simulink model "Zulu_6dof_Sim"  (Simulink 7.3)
settings: Solver=ode45  StartTime=0.0  StopTime=315  RelTol=1e-4
InitFcn:
  | init
StopFcn:
  | pl
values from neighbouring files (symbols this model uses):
  accel = [-225, 0, 0]    [init.m]
  ch = 7.761    [init.m]
  d2r = pi/180    (= 0.0174532925199)    [init.m]    (also in pl.m; run.m; LQR_Des.m)
  Euler_0 = [0, 49.766, 0]*d2r    [init.m]
  h0 = 43031    [init.m]
  Ixxpr = ee*Zulu_Mass(:,2)    [init.m]
  Ixypr = ee*Zulu_Mass(:,5)    [init.m]
  Ixzpr = ee*Zulu_Mass(:,6)    [init.m]
  Iyypr = ee*Zulu_Mass(:,3)    [init.m]
  Iyzpr = ee*Zulu_Mass(:,7)    [init.m]
  Izzpr = ee*Zulu_Mass(:,4)    [init.m]
  mrc = [x_ref, y_ref, z_ref]    [init.m]
  msspr = ee*Zulu_Mass(:,1)    [init.m]
  r2d = 180/pi    (= 57.2957795131)    [init.m]    (also in pl.m; run.m; LQR_Des.m)
  rcs1 = [-120.0, -4.0, -0.0]    [init.m]
  rcs2 = [-120.0, +4.0, -0.0]    [init.m]
  sp = 7.761    [init.m]
  Sref = 47.308    [init.m]
  Tst2 = 170.0    (= 170)    [init.m]
  Tstg = 91.2    [init.m]
  tvc1 = [-244.6, -8.7, 0.0]    [init.m]
  tvc2 = [-244.6, +8.7, 0.0]    [init.m]
  tvc3 = [-244.6,  0.0, 0.0]    [init.m]
  tvc4 = [-200.0, 0.0, 0.06]    [init.m]
  Xcgpr = ee*Zulu_Mass(:,8)    [init.m]
  Ycgpr = ee*Zulu_Mass(:,9)    [init.m]
  Zcgpr = ee*Zulu_Mass(:,10)    [init.m]
undefined symbols (not defined in the file or in its folder): Cl, Cl2, Cm, Cm2, Cn, Cn2, Continuous, CX, CX2, CY, CY2, CZ, CZ2, Dryden, Earth, F, ft, km, Light, MIL, q, r, sigbuilder_block, STD, WGS84
libraries: aerolibutil x7, aerolibasang x3, aerolibwind2 x3, aerolibactuator x2, aerolibconvert2 x1, aerolibatmos2 x1, aerolibgravity2 x1, aerolibadyn x1, aerolib6dof2 x1
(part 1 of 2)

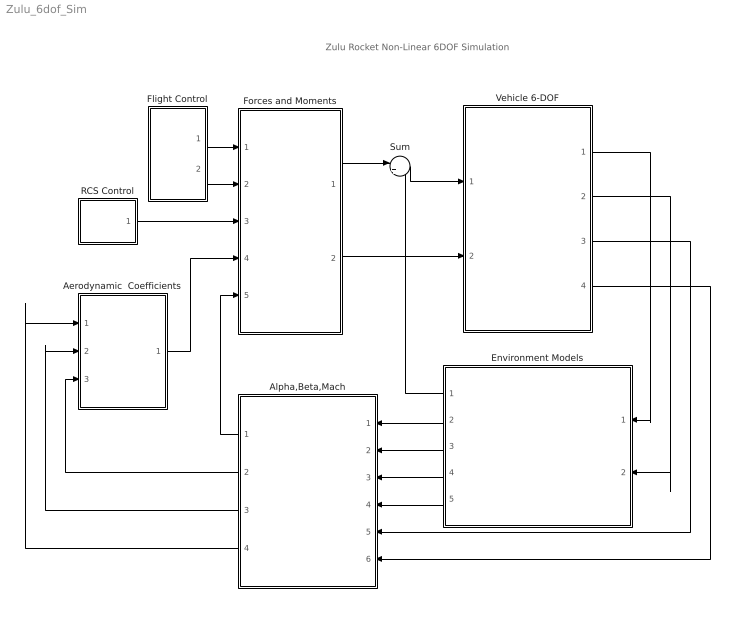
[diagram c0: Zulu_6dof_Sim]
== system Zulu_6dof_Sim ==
  note: Zulu Rocket Non-Linear 6DOF Simulation
  Aerodynamic  Coefficients : Subsystem
  Alpha,Beta,Mach : Subsystem
  Environment Models : Subsystem
  Flight Control : Subsystem
  Forces and Moments : Subsystem
  RCS Control : Subsystem
  Sum : Sum  Inputs=|++  OutDataType=sfix(16)  OutScaling=2^0
  Vehicle 6-DOF : Subsystem
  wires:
  Vehicle 6-DOF/3(Vb) -> Alpha,Beta,Mach/5(Vb)
  Vehicle 6-DOF/1(Ve) -> Environment Models/1(Ve)
  Forces and Moments/1(X,Y,Z) -> Sum/1
  Environment Models/2(Speed of Sound) -> Alpha,Beta,Mach/1(Speed of Sound)
  Environment Models/3(Wind Velocity) -> Alpha,Beta,Mach/2(Wind Velocity)
  Environment Models/4(Air Density) -> Alpha,Beta,Mach/3(Air Density)
  Environment Models/5(Wind Angular Rates) -> Alpha,Beta,Mach/4(Wind Angul Rates)
  Environment Models/1(Fgrv) -> Sum/2
  Alpha,Beta,Mach/4(Incid) -> Aerodynamic  Coefficients/1(Incid)
  Alpha,Beta,Mach/3(Mach) -> Aerodynamic  Coefficients/2(Mach)
  Vehicle 6-DOF/4(w) -> Alpha,Beta,Mach/6("p,q,r ")
  Alpha,Beta,Mach/1(qbar) -> Forces and Moments/5(qbar)
  Sum/1 -> Vehicle 6-DOF/1(Fxyz)
  Forces and Moments/2(LMN) -> Vehicle 6-DOF/2(Mxyz)
  Aerodynamic  Coefficients/1(Coeff) -> Forces and Moments/4(Coeff)
  RCS Control/1(Th_Cmd) -> Forces and Moments/3(Th_rcs)
  Flight Control/2(DZ) -> Forces and Moments/2(DZ)
  Flight Control/1(DY) -> Forces and Moments/1(DY)
  Vehicle 6-DOF/2(Height) -> Environment Models/2(Height)
  Alpha,Beta,Mach/2(pqr_w) -> Aerodynamic  Coefficients/3(p,q,r)

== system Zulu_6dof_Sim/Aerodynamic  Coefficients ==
  note: Aero Coefficients funct. of: Alpha, Beta, Mach#
  Incid : Inport  OutDataType=sfix(16)  OutScaling=2^0
  Mach : Inport  Port=2  OutDataType=sfix(16)  OutScaling=2^0
  p,q,r : Inport  Port=3  OutDataType=sfix(16)  OutScaling=2^0
  Angle Conversion : aerolibconvert2/Angle Conversion  SystemSampleTime=-1  IU=rad  OU=deg
  Clock : Clock
  Damping Coefficients : Subsystem
  Stage-1 Aero  Coefficients : Subsystem
  Stage-2 Aero  Coefficients : Subsystem
  Sum1 : Sum  Inputs=|++  OutDataType=fixdt(1, 16)  OutScaling=2^0
  Switch : Switch  Threshold=Tstg  OutDataType=fixdt(1, 16)  OutScaling=2^0
  Coeff : Outport  OutDataType=sfix(16)  OutScaling=2^0  InitialOutput=0
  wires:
  Incid/1 -> Angle Conversion/1
  Angle Conversion/1 -> Stage-1 Aero  Coefficients/1(albet), Stage-2 Aero  Coefficients/1(albet), Damping Coefficients/1(albet)
  Mach/1 -> Stage-1 Aero  Coefficients/2(Mach), Stage-2 Aero  Coefficients/2(Mach)
  Clock/1 -> Switch/2
  Stage-2 Aero  Coefficients/1(Coeff) -> Switch/1
  Switch/1 -> Coeff/1
  p,q,r/1 -> Damping Coefficients/3(p,q,r)
  [Vo] -> Damping Coefficients/2(V)
  Stage-1 Aero  Coefficients/1(Coeff) -> Sum1/1
  Sum1/1 -> Switch/3
  Damping Coefficients/1(cl) -> Sum1/2

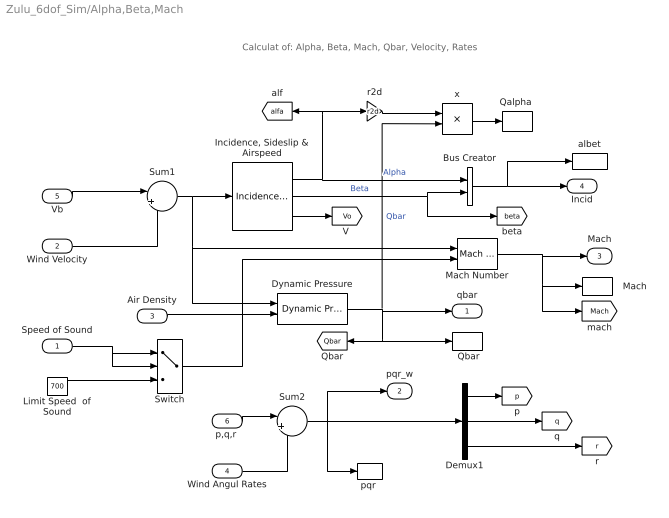
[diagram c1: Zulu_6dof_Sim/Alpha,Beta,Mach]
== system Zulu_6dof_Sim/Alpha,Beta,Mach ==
  note: Calculat of: Alpha, Beta, Mach, Qbar, Velocity, Rates
  Speed of Sound : Inport  OutDataType=sfix(16)  OutScaling=2^0
  Wind Velocity : Inport  Port=2  PortDimensions=3  OutDataType=sfix(16)  OutScaling=2^0
  Air Density : Inport  Port=3  OutDataType=sfix(16)  OutScaling=2^0
  Wind Angul Rates : Inport  Port=4  PortDimensions=3  OutDataType=sfix(16)  OutScaling=2^0
  Vb : Inport  Port=5  PortDimensions=3  OutDataType=sfix(16)  OutScaling=2^0
  "p,q,r " : Inport  Port=6  PortDimensions=3  OutDataType=sfix(16)  OutScaling=2^0
  "  Mach" : ToWorkspace  VariableName=Mach  SampleTime=-1  SaveFormat=Array
  " Qbar" : ToWorkspace  VariableName=Qbar  SampleTime=-1  SaveFormat=Array
  Bus Creator : BusCreator  Inputs=2
  Demux1 : Demux  Outputs=3
  Dynamic Pressure : aerolibasang/Dynamic Pressure  SystemSampleTime=-1
  "Incidence, Sideslip & Airspeed" : aerolibasang/Incidence, Sideslip, & Airspeed  SystemSampleTime=-1
  Limit Speed  of Sound : Constant  Value=700  OutDataType=fixdt(1, 16)  OutScaling=2^0
  Mach Number : aerolibasang/Mach Number  SystemSampleTime=-1
  "Qalpha " : ToWorkspace  VariableName=Qalfa  SampleTime=-1  SaveFormat=Array
  Sum1 : Sum  Inputs=|+-  OutDataType=sfix(16)  OutScaling=2^0
  Sum2 : Sum  Inputs=|++  OutDataType=sfix(16)  OutScaling=2^0
  Switch : Switch  Threshold=700  OutDataType=fixdt(1, 16)  OutScaling=2^0
  albet : ToWorkspace  VariableName=albet  SampleTime=-1  SaveFormat=Array
  "pqr " : ToWorkspace  VariableName=pqr  SampleTime=-1  SaveFormat=Array
  r2d : Gain  Gain=r2d  ParameterDataType=sfix(16)  ParameterScaling=2^0  OutDataType=sfix(16)  OutScaling=2^0
  x : Product  OutDataType=fixdt(1, 16)  OutScaling=2^0
  qbar : Outport  OutDataType=sfix(16)  OutScaling=2^0  InitialOutput=0
  pqr_w : Outport  Port=2  OutDataType=sfix(16)  OutScaling=2^0
  Mach : Outport  Port=3  OutDataType=sfix(16)  OutScaling=2^0
  Incid : Outport  Port=4  OutDataType=sfix(16)  OutScaling=2^0
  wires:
  "Incidence, Sideslip & Airspeed"/3 -> [Vo]
  Dynamic Pressure/1 -> qbar/1, " Qbar"/1, [Qbar], x/2  "Qbar"
  Mach Number/1 -> Mach/1, "  Mach"/1, [Mach]
  Sum1/1 -> Dynamic Pressure/1, Mach Number/1, "Incidence, Sideslip & Airspeed"/1
  Vb/1 -> Sum1/1
  Speed of Sound/1 -> Switch/1, Switch/2
  Wind Velocity/1 -> Sum1/2
  "Incidence, Sideslip & Airspeed"/2 -> Bus Creator/2, [beta]  "Beta"
  Bus Creator/1 -> Incid/1, albet/1
  "Incidence, Sideslip & Airspeed"/1 -> Bus Creator/1, [alfa], r2d/1  "Alpha"
  "p,q,r "/1 -> Sum2/1
  Sum2/1 -> Demux1/1, "pqr "/1, pqr_w/1
  Demux1/2 -> [q]
  Demux1/3 -> [r]
  Demux1/1 -> [p]
  Air Density/1 -> Dynamic Pressure/2
  Switch/1 -> Mach Number/2
  Limit Speed  of Sound/1 -> Switch/3
  Wind Angul Rates/1 -> Sum2/2
  x/1 -> "Qalpha "/1
  r2d/1 -> x/1

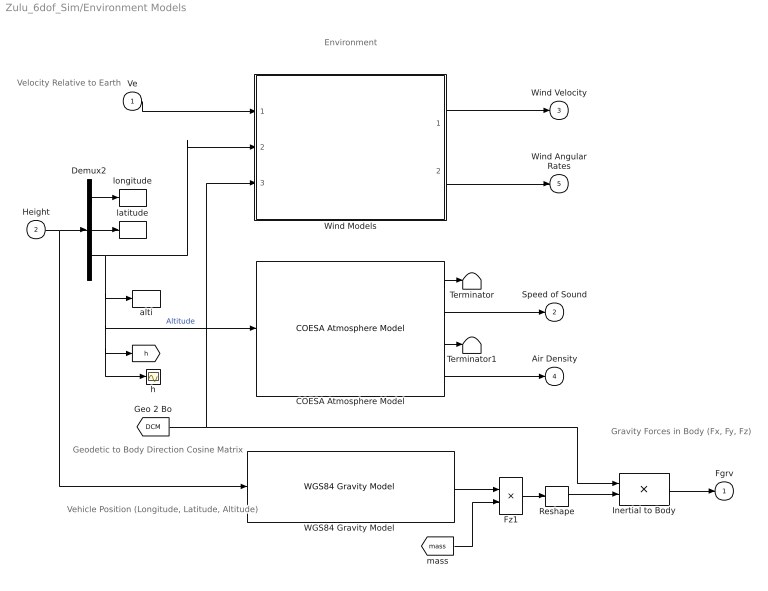
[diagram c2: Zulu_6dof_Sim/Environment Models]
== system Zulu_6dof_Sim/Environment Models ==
  note: Gravity Forces in Body (Fx, Fy, Fz)
  note: Environment
  note: Geodetic to Body Direction Cosine Matrix
  note: Vehicle Position (Longitude, Latitude, Altitude)
  note: Velocity Relative to Earth
  Ve : Inport  OutDataType=sfix(16)  OutScaling=2^0
  Height : Inport  Port=2  OutDataType=sfix(16)  OutScaling=2^0
  COESA Atmosphere Model : aerolibatmos2/COESA Atmosphere Model  SystemSampleTime=-1  units=English (Velocity in ft/s)  spec=MIL-STD-210C  model=Profile  profile_var=Low density  profile_percent=1%  profile_alt=5 km (16404 ft)  envelope_var=High temperature  envelope_percent=1%  action=Warning
  Demux2 : Demux  Outputs=3
  Fz1 : Product  OutDataType=fixdt(1, 16)  OutScaling=2^0
  Inertial to Body : Product  Multiplication=Matrix(*)  OutDataType=sfix(16)  OutScaling=2^0
  Reshape : Reshape
  Terminator : Terminator
  Terminator1 : Terminator
  "WGS84 Gravity Model " : aerolibgravity2/WGS84 Gravity Model   SystemSampleTime=-1  model=WGS84 Taylor Series  units=English  no_atmos=on  precessing=on  jd_loc=off  month=October  day=10  year=2004  no_centrifugal=on  action=None
  Wind Models : Subsystem
  alti : ToWorkspace  VariableName=alti  SampleTime=-1  SaveFormat=Array
  h : Scope
  latitude : ToWorkspace  VariableName=latit  SampleTime=-1  SaveFormat=Array
  longitude : ToWorkspace  VariableName=long  SampleTime=-1  SaveFormat=Array
  Fgrv : Outport  OutDataType=sfix(16)  OutScaling=2^0  InitialOutput=0
  Speed of Sound : Outport  Port=2  OutDataType=sfix(16)  OutScaling=2^0  InitialOutput=0
  Wind Velocity : Outport  Port=3  OutDataType=sfix(16)  OutScaling=2^0  InitialOutput=0
  Air Density : Outport  Port=4  OutDataType=sfix(16)  OutScaling=2^0  InitialOutput=0
  Wind Angular Rates : Outport  Port=5  OutDataType=sfix(16)  OutScaling=2^0  InitialOutput=0
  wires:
  Reshape/1 -> Inertial to Body/2
  "WGS84 Gravity Model "/1 -> Fz1/1
  Fz1/1 -> Reshape/1
  COESA Atmosphere Model/1 -> Terminator/1
  COESA Atmosphere Model/2 -> Speed of Sound/1
  COESA Atmosphere Model/3 -> Terminator1/1
  COESA Atmosphere Model/4 -> Air Density/1
  [DCM] -> Inertial to Body/1, Wind Models/3(DCM)
  Inertial to Body/1 -> Fgrv/1
  Wind Models/2(pg,qg,rg) -> Wind Angular Rates/1
  Ve/1 -> Wind Models/1(Ve)
  Wind Models/1(ug,vg,wg) -> Wind Velocity/1
  [mass] -> Fz1/2
  Demux2/3 -> alti/1, COESA Atmosphere Model/1, [h], h/1, Wind Models/2(Altitude)  "Altitude"
  Demux2/1 -> longitude/1
  Demux2/2 -> latitude/1
  Height/1 -> Demux2/1, "WGS84 Gravity Model "/1

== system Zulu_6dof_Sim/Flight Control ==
  note: Pitch Gimbal Deflections
  note: Yaw Gimbal Deflections
  note: Flight Control System
  note: Engine Mount Angles
  "DY " : ToWorkspace  VariableName=DY  SampleTime=-1  SaveFormat=Array
  DY0 : Constant  Value=[0.7, 0.7, 0]*d2r  OutDataType=fixdt(1, 16)  OutScaling=2^0
  "DZ " : ToWorkspace  VariableName=DZ  SampleTime=-1  SaveFormat=Array
  Lateral FCS : Subsystem
  Nonlinear Actuator : aerolibactuator/Second Order Nonlinear Actuator  SystemSampleTime=-1  wn_fin=65  z_fin=0.7  fin_max=5*pi/180  fin_min=-5*pi/180  fin_maxrate=25*pi/180  fin_act_0=0
  "Nonlinear Actuator " : aerolibactuator/Second Order Nonlinear Actuator  SystemSampleTime=-1  wn_fin=65  z_fin=0.7  fin_max=5*pi/180  fin_min=-5*pi/180  fin_maxrate=25*pi/180  fin_act_0=0
  Pitch FCS : Subsystem
  Sum : Sum  Inputs=|++  OutDataType=fixdt(1, 16)  OutScaling=2^0
  Sum1 : Sum  Inputs=++|  OutDataType=fixdt(1, 16)  OutScaling=2^0
  DY : Outport
  DZ : Outport  Port=2
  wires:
  Pitch FCS/1(DY) -> Sum/1
  Sum/1 -> Nonlinear Actuator/1
  "Nonlinear Actuator "/1 -> DZ/1, "DZ "/1, [DZ]
  Lateral FCS/1(DY) -> Sum/2
  Lateral FCS/2(DZ) -> "Nonlinear Actuator "/1
  Nonlinear Actuator/1 -> Sum1/2
  DY0/1 -> Sum1/1
  Sum1/1 -> DY/1, "DY "/1, [DY]

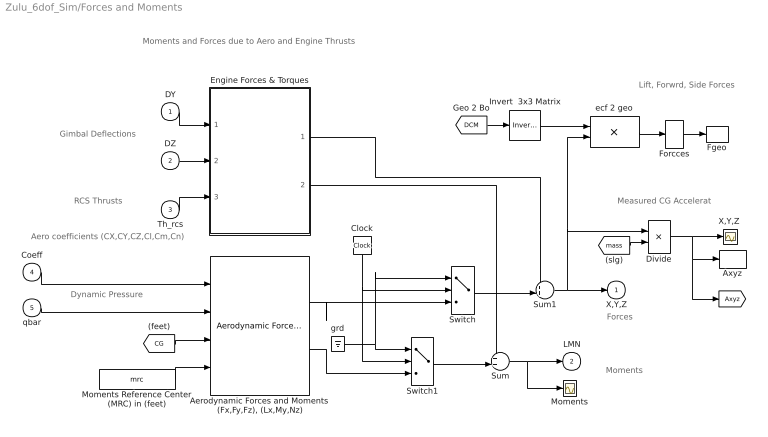
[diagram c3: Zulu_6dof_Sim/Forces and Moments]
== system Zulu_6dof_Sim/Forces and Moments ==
  note: Gimbal Deflections
  note: Moments and Forces due to Aero and Engine Thrusts
  note: Dynamic Pressure
  note: Aero coefficients (CX,CY,CZ,Cl,Cm,Cn)
  note: RCS Thrusts
  note: Forces
  note: Measured CG Accelerat
  note: Moments
  note: Lift, Forwrd, Side Forces
  DY : Inport  OutDataType=sfix(16)  OutScaling=2^0
  DZ : Inport  Port=2  OutDataType=sfix(16)  OutScaling=2^0
  Th_rcs : Inport  Port=3  OutDataType=sfix(16)  OutScaling=2^0
  Coeff : Inport  Port=4  OutDataType=sfix(16)  OutScaling=2^0
  qbar : Inport  Port=5  OutDataType=sfix(16)  OutScaling=2^0
  "Aerodynamic Forces and Moments (Fx,Fy,Fz), (Lx,My,Nz)" : aerolibadyn/Aerodynamic Forces and Moments   SystemSampleTime=-1  inputAxes=Body  outputForceAxes=Body  outputMomentAxes=Body  S=Sref  b=sp  cbar=ch
  Axyz : ToWorkspace  VariableName=Axyz  SampleTime=-1  SaveFormat=Array
  Clock : Clock
  Divide : Product  Inputs=*/  OutDataType=fixdt(1, 16)  OutScaling=2^-10
  Engine Forces & Torques : Subsystem
  Fgeo : ToWorkspace  VariableName=Flds  SampleTime=-1  SaveFormat=Array
  Forcces : Selector  InputPortWidth=3  IndexOptions=Index vector (dialog)  Indices=[3,1,2]  OutputSizes=1
  Invert  3x3 Matrix : aerolibutil/Invert  3x3 Matrix  SystemSampleTime=-1
  Moments : Scope
  Moments Reference Center (MRC) in (feet) : Constant  Value=mrc  OutDataType=sfix(16)  OutScaling=2^0
  Sum : Sum  Inputs=++|  OutDataType=fixdt(1, 16)  OutScaling=2^0
  Sum1 : Sum  Inputs=++|  OutDataType=sfix(16)  OutScaling=2^0
  Switch : Switch  Threshold=Tst2  OutDataType=fixdt(1, 16)  OutScaling=2^0
  Switch1 : Switch  Threshold=Tst2  OutDataType=fixdt(1, 16)  OutScaling=2^0
  "X,Y,Z " : Scope
  ecf 2 geo : Product  Multiplication=Matrix(*)  OutDataType=sfix(16)  OutScaling=2^0
  grd : Ground
  X,Y,Z : Outport  OutDataType=sfix(16)  OutScaling=2^0  InitialOutput=0
  LMN : Outport  Port=2  OutDataType=sfix(16)  OutScaling=2^0  InitialOutput=0
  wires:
  Engine Forces & Torques/1(Force) -> Sum1/1
  Engine Forces & Torques/2(Torqu) -> Sum/1
  DY/1 -> Engine Forces & Torques/1(DY (rad))
  DZ/1 -> Engine Forces & Torques/2(DZ (rad))
  Sum/1 -> LMN/1, Moments/1
  Forcces/1 -> Fgeo/1
  Divide/1 -> "X,Y,Z "/1, Axyz/1, [Axyz]
  Moments Reference Center (MRC) in (feet)/1 -> "Aerodynamic Forces and Moments (Fx,Fy,Fz), (Lx,My,Nz)"/4
  Sum1/1 -> X,Y,Z/1, Divide/1, ecf 2 geo/2
  qbar/1 -> "Aerodynamic Forces and Moments (Fx,Fy,Fz), (Lx,My,Nz)"/2
  Coeff/1 -> "Aerodynamic Forces and Moments (Fx,Fy,Fz), (Lx,My,Nz)"/1
  [mass] -> Divide/2
  [CG] -> "Aerodynamic Forces and Moments (Fx,Fy,Fz), (Lx,My,Nz)"/3
  Th_rcs/1 -> Engine Forces & Torques/3(Th_rcs)
  Switch/1 -> Sum1/2
  Switch1/1 -> Sum/2
  Clock/1 -> Switch/2, Switch1/2
  "Aerodynamic Forces and Moments (Fx,Fy,Fz), (Lx,My,Nz)"/2 -> Switch1/3
  "Aerodynamic Forces and Moments (Fx,Fy,Fz), (Lx,My,Nz)"/1 -> Switch/3
  grd/1 -> Switch1/1, Switch/1
  ecf 2 geo/1 -> Forcces/1
  Invert  3x3 Matrix/1 -> ecf 2 geo/1
  [DCM] -> Invert  3x3 Matrix/1

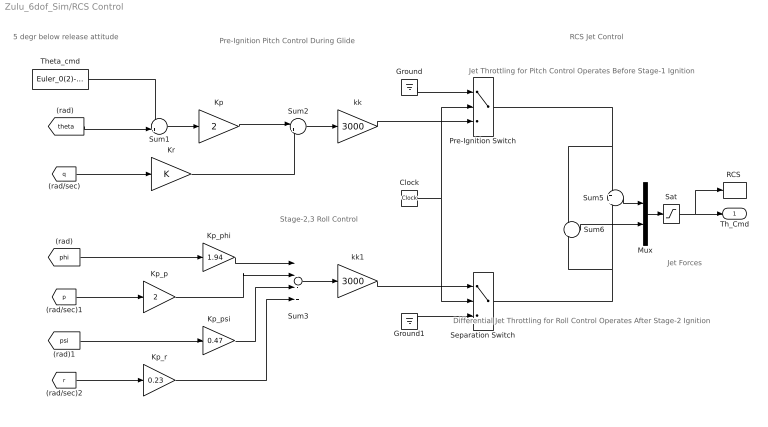
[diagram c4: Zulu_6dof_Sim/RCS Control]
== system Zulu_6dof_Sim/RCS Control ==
  note: Pre-Ignition Pitch Control During Glide
  note: 5 degr below release attitude
  note: Stage-2,3 Roll Control
  note: Jet Forces
  note: RCS Jet Control
  note: Jet Throttling for Pitch Control Operates Before Stage-1 Ignition
  note: Differential Jet Throttling for Roll Control Operates After Stage-2 Ignition
  Clock : Clock
  Ground : Ground
  Ground1 : Ground
  Kp : Gain  Gain=2  ParameterDataType=sfix(16)  ParameterScaling=2^0  OutDataType=sfix(16)  OutScaling=2^0
  Kp_p : Gain  Gain=2  ParameterDataType=sfix(16)  ParameterScaling=2^0  OutDataType=sfix(16)  OutScaling=2^0
  Kp_phi : Gain  Gain=1.94  ParameterDataType=sfix(16)  ParameterScaling=2^0  OutDataType=sfix(16)  OutScaling=2^0
  Kp_psi : Gain  Gain=0.47  ParameterDataType=sfix(16)  ParameterScaling=2^0  OutDataType=sfix(16)  OutScaling=2^0
  Kp_r : Gain  Gain=0.23  ParameterDataType=sfix(16)  ParameterScaling=2^0  OutDataType=sfix(16)  OutScaling=2^0
  Kr : Gain  ParameterDataType=sfix(16)  ParameterScaling=2^0  OutDataType=sfix(16)  OutScaling=2^0
  Mux : Mux  Inputs=2
  Pre-Ignition Switch : Switch  Threshold=4.5  OutDataType=fixdt(1, 16)  OutScaling=2^0
  "RCS " : ToWorkspace  VariableName=RCS  SampleTime=-1  SaveFormat=Array
  Sat : Saturate  UpperLimit=800  LowerLimit=-800  OutDataType=fixdt(1, 16)  OutScaling=2^0
  Separation Switch : Switch  Threshold=Tstg  OutDataType=fixdt(1, 16)  OutScaling=2^0
  Sum1 : Sum  Inputs=-+|  OutDataType=fixdt(1, 16)  OutScaling=2^0
  Sum2 : Sum  Inputs=|++  OutDataType=fixdt(1, 16)  OutScaling=2^0
  Sum3 : Sum  Inputs=++-+  OutDataType=fixdt(1, 16)  OutScaling=2^0
  Sum5 : Sum  Inputs=+|+  OutDataType=fixdt(1, 16)  OutScaling=2^0
  Sum6 : Sum  Inputs=+|-  OutDataType=fixdt(1, 16)  OutScaling=2^0
  Theta_cmd : Constant  Value=Euler_0(2)-6.2*d2r  OutDataType=fixdt(1, 16)  OutScaling=2^0
  kk : Gain  Gain=3000  ParameterDataType=sfix(16)  ParameterScaling=2^0  OutDataType=sfix(16)  OutScaling=2^0
  kk1 : Gain  Gain=3000  ParameterDataType=sfix(16)  ParameterScaling=2^0  OutDataType=sfix(16)  OutScaling=2^0
  Th_Cmd : Outport
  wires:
  [theta] -> Sum1/2
  Theta_cmd/1 -> Sum1/1
  Sum1/1 -> Kp/1
  [q] -> Kr/1
  Kp/1 -> Sum2/1
  Kr/1 -> Sum2/2
  Sum2/1 -> kk/1
  kk/1 -> Pre-Ignition Switch/3
  Pre-Ignition Switch/1 -> Sum5/1, Sum6/1
  Ground/1 -> Pre-Ignition Switch/1
  Mux/1 -> Sat/1
  [phi] -> Kp_phi/1
  [p] -> Kp_p/1
  Sum3/1 -> kk1/1
  kk1/1 -> Separation Switch/1
  Ground1/1 -> Separation Switch/3
  Sum5/1 -> Mux/1
  Sum6/1 -> Mux/2
  Separation Switch/1 -> Sum5/2, Sum6/2
  Clock/1 -> Pre-Ignition Switch/2, Separation Switch/2
  Sat/1 -> Th_Cmd/1, "RCS "/1
  [r] -> Kp_r/1
  [psi] -> Kp_psi/1
  Kp_psi/1 -> Sum3/3
  Kp_r/1 -> Sum3/4
  Kp_p/1 -> Sum3/2
  Kp_phi/1 -> Sum3/1

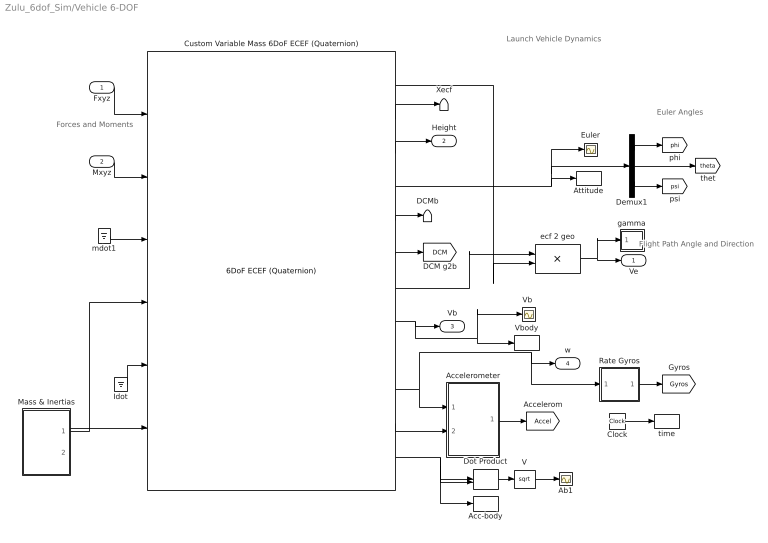
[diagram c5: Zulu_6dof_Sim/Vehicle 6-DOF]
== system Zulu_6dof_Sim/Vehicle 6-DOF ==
  note: Flight Path Angle and Direction
  note: Euler Angles
  note: Forces and Moments
  note: Launch Vehicle Dynamics
  Fxyz : Inport
  Mxyz : Inport  Port=2
  Ab1 : Scope
  Acc-body : ToWorkspace  VariableName=Ab  SampleTime=-1  SaveFormat=Array
  Accelerometer : Subsystem
  Attitude : ToWorkspace  VariableName=Euler  SampleTime=-1  SaveFormat=Array
  Clock : Clock
  Custom Variable Mass 6DoF ECEF (Quaternion) : aerolib6dof2/6DoF ECEF (Quaternion)  SystemSampleTime=-1  units=English (Velocity in ft/s)  mtype=Custom Variable  xg_0=[0 0 h0]  Vm_0=Uvw_0  eul_0=Euler_0  pm_0=pqr_0  mass_0=1.0  mass_e=0.5  mass_f=2.0  inertia=eye(3)  inertia_e=eye(3)  inertia_f=2*eye(3)  ptype=Earth (WGS84)  F=1/298.257223563  R=20925646.3255  w_E=7292115e-11  angle_in=Internal  LG0=0
  DCMb : Terminator
  Demux1 : Demux  Outputs=3
  Dot Product : DotProduct  OutDataType=sfix(16)  OutScaling=2^-10  SaturateOnIntegerOverflow=on
  Euler : Scope
  Idot : Ground
  Mass & Inertias : Subsystem
  Rate Gyros : Subsystem
  V : Math  Operator=sqrt  OutDataType=sfix(16)  OutScaling=2^0
  "Vb " : Scope
  Vbody : ToWorkspace  VariableName=Vb  SampleTime=-1  SaveFormat=Array
  Xecf : Terminator
  ecf 2 geo : Product  Multiplication=Matrix(*)  OutDataType=sfix(16)  OutScaling=2^0
  gamma : Subsystem
  mdot1 : Ground
  time : ToWorkspace  VariableName=time  SampleTime=-1  SaveFormat=Array
  Ve : Outport
  Height : Outport  Port=2
  Vb : Outport  Port=3
  w : Outport  Port=4
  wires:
  Mass & Inertias/2(Inert) -> Custom Variable Mass 6DoF ECEF (Quaternion)/6
  Mass & Inertias/1(mass) -> Custom Variable Mass 6DoF ECEF (Quaternion)/4
  Fxyz/1 -> Custom Variable Mass 6DoF ECEF (Quaternion)/1
  Mxyz/1 -> Custom Variable Mass 6DoF ECEF (Quaternion)/2
  Dot Product/1 -> V/1
  mdot1/1 -> Custom Variable Mass 6DoF ECEF (Quaternion)/3
  V/1 -> Ab1/1
  Demux1/2 -> [theta]
  Demux1/1 -> [phi]
  Demux1/3 -> [psi]
  Custom Variable Mass 6DoF ECEF (Quaternion)/7 -> ecf 2 geo/1
  Idot/1 -> Custom Variable Mass 6DoF ECEF (Quaternion)/5
  Custom Variable Mass 6DoF ECEF (Quaternion)/1 -> ecf 2 geo/2
  Custom Variable Mass 6DoF ECEF (Quaternion)/3 -> Height/1
  ecf 2 geo/1 -> Ve/1, gamma/1(Ve)
  Custom Variable Mass 6DoF ECEF (Quaternion)/8 -> Vb/1, Vbody/1, "Vb "/1
  Custom Variable Mass 6DoF ECEF (Quaternion)/10 -> w/1, Rate Gyros/1(w), Accelerometer/1(w)
  Custom Variable Mass 6DoF ECEF (Quaternion)/11 -> Accelerometer/2(wdot)
  Custom Variable Mass 6DoF ECEF (Quaternion)/4 -> Attitude/1, Demux1/1, Euler/1
  Custom Variable Mass 6DoF ECEF (Quaternion)/2 -> Xecf/1
  Custom Variable Mass 6DoF ECEF (Quaternion)/5 -> DCMb/1
  Clock/1 -> time/1
  Custom Variable Mass 6DoF ECEF (Quaternion)/6 -> [DCM]
  Accelerometer/1(Accel) -> [Accel]
  Rate Gyros/1(Gyro) -> [Gyros]
  Custom Variable Mass 6DoF ECEF (Quaternion)/12 -> Dot Product/1, Dot Product/2, Acc-body/1

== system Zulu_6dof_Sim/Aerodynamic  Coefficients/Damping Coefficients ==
  albet : Inport  OutDataType=sfix(16)  OutScaling=2^0
  V : Inport  Port=2  OutDataType=sfix(16)  OutScaling=2^0
  p,q,r : Inport  Port=3  OutDataType=sfix(16)  OutScaling=2^0
  Alpha Lookup : PreLookup  BreakpointsData=Alfa2  BeginIndexSearchUsingPreviousIndexResult=on  ProcessOutOfRangeInput=Linear extrapolation  IndexDataType=sfix(16)  FractionDataType=sfix(16)  FractionScaling=2^0
  Bus Creator : BusCreator  Inputs=2
  Demux : Demux  Outputs=3
  Demux1 : Demux  Outputs=2
  Product : Product  OutDataType=sfix(16)  OutScaling=2^0
  Product1 : Product  OutDataType=sfix(16)  OutScaling=2^0
  Product2 : Product  OutDataType=sfix(16)  OutScaling=2^0
  Product3 : Product  Inputs=*/  OutDataType=sfix(16)  OutScaling=2^0
  Reference Length : Gain  Gain=ch/2  ParameterDataType=sfix(16)  ParameterScaling=2^0  OutDataType=sfix(16)  OutScaling=2^0
  Reference Span : Gain  Gain=sp/2  ParameterDataType=sfix(16)  ParameterScaling=2^0  OutDataType=sfix(16)  OutScaling=2^0
  "Reference Span " : Gain  Gain=sp/2  ParameterDataType=sfix(16)  ParameterScaling=2^0  OutDataType=sfix(16)  OutScaling=2^0
  Sum1 : Sum  Inputs=+++  OutDataType=sfix(16)  OutScaling=2^0
  beta : Terminator
  p : Subsystem
  q : Subsystem
  r : Subsystem
  cl : Outport  OutDataType=sfix(16)  OutScaling=2^0  InitialOutput=0
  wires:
  p,q,r/1 -> Demux/1
  Demux/1 -> Product/2  "p"
  Demux/2 -> Product1/2  "q"
  Demux/3 -> Product2/2  "r"
  r/1(C) -> Product2/1
  q/1(C) -> Product1/1
  p/1(C) -> Product/1
  Bus Creator/1 -> r/1(Alpha), q/1(Alpha), p/1(Alpha)
  Alpha Lookup/1 -> Bus Creator/1  "k"
  Alpha Lookup/2 -> Bus Creator/2  "f"
  Sum1/1 -> Product3/1
  V/1 -> Product3/2
  Product3/1 -> cl/1
  Product1/1 -> Reference Length/1
  Product2/1 -> "Reference Span "/1
  Product/1 -> Reference Span/1
  Reference Length/1 -> Sum1/2
  Reference Span/1 -> Sum1/1
  "Reference Span "/1 -> Sum1/3
  albet/1 -> Demux1/1
  Demux1/1 -> Alpha Lookup/1
  Demux1/2 -> beta/1

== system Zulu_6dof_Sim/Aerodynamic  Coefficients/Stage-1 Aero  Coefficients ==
  albet : Inport  OutDataType=sfix(16)  OutScaling=2^0
  Mach : Inport  Port=2  OutDataType=sfix(16)  OutScaling=2^0
  " CA" : Scope
  " CZ" : Scope
  " Cl" : Scope
  " Cm" : Scope
  " Cn" : Scope
  " Cy" : Scope
  Alpha Lookup : PreLookup  BreakpointsData=Alfas  BeginIndexSearchUsingPreviousIndexResult=on  ProcessOutOfRangeInput=Linear extrapolation  IndexDataType=sfix(16)  FractionDataType=sfix(16)  FractionScaling=2^0
  Beta Lookup : PreLookup  BreakpointsData=Betas  BeginIndexSearchUsingPreviousIndexResult=on  ProcessOutOfRangeInput=Linear extrapolation  IndexDataType=sfix(16)  FractionDataType=sfix(16)  FractionScaling=2^0
  CX : Interpolation_n-D  NumberOfTableDimensions=3  Table=CX  CheckIndexInCode=off  OutDataType=sfix(16)  OutScaling=2^0
  CY : Interpolation_n-D  NumberOfTableDimensions=3  Table=CY  CheckIndexInCode=off  OutDataType=sfix(16)  OutScaling=2^0
  CZ : Interpolation_n-D  NumberOfTableDimensions=3  Table=CZ  CheckIndexInCode=off  OutDataType=sfix(16)  OutScaling=2^0
  Cl : Interpolation_n-D  NumberOfTableDimensions=3  Table=Cl  CheckIndexInCode=off  OutDataTypeMode=double  OutDataType=sfix(16)  OutScaling=2^0  OutDataTypeStr=double
  Cm : Interpolation_n-D  NumberOfTableDimensions=3  Table=Cm  CheckIndexInCode=off  OutDataType=sfix(16)  OutScaling=2^0
  Cn : Interpolation_n-D  NumberOfTableDimensions=3  Table=Cn  CheckIndexInCode=off  OutDataType=sfix(16)  OutScaling=2^0
  Demux : Demux  Outputs=2
  Mach Lookup : PreLookup  BreakpointsData=Machs  BeginIndexSearchUsingPreviousIndexResult=on  ProcessOutOfRangeInput=Linear extrapolation  IndexDataType=sfix(16)  FractionDataType=sfix(16)  FractionScaling=2^0
  Mux1 : Mux  Inputs=6
  Coeff : Outport  OutDataType=sfix(16)  OutScaling=2^0  InitialOutput=0
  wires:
  Demux/1 -> Alpha Lookup/1
  CX/1 -> Mux1/1, " CA"/1
  CY/1 -> Mux1/2, " Cy"/1
  CZ/1 -> Mux1/3, " CZ"/1
  Cl/1 -> Mux1/4, " Cl"/1
  Cm/1 -> Mux1/5, " Cm"/1
  Cn/1 -> Mux1/6, " Cn"/1
  Alpha Lookup/1 -> CX/1, CY/1, Cm/1, Cn/1, Cl/1, CZ/1
  Alpha Lookup/2 -> CX/2, CY/2, CZ/2, Cl/2, Cm/2, Cn/2
  Mach Lookup/1 -> CY/3, Cm/3, Cn/3, Cl/3, CZ/3, CX/3
  Mach Lookup/2 -> CY/4, Cm/4, Cn/4, Cl/4, CZ/4, CX/4
  Beta Lookup/1 -> CX/5, Cm/5, Cn/5, Cl/5, CZ/5, CY/5
  Beta Lookup/2 -> CX/6, CY/6, Cm/6, Cn/6, Cl/6, CZ/6
  Demux/2 -> Beta Lookup/1
  albet/1 -> Demux/1
  Mach/1 -> Mach Lookup/1
  Mux1/1 -> Coeff/1

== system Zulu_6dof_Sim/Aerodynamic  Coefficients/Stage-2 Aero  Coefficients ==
  albet : Inport  OutDataType=sfix(16)  OutScaling=2^0
  Mach : Inport  Port=2  OutDataType=sfix(16)  OutScaling=2^0
  " CA" : Scope
  " CZ" : Scope
  " Cl" : Scope
  " Cm" : Scope
  " Cn" : Scope
  " Cy" : Scope
  Alpha Lookup : PreLookup  BreakpointsData=Alfa2  BeginIndexSearchUsingPreviousIndexResult=on  ProcessOutOfRangeInput=Linear extrapolation  IndexDataType=sfix(16)  FractionDataType=sfix(16)  FractionScaling=2^0
  Beta Lookup : PreLookup  BreakpointsData=Betas  BeginIndexSearchUsingPreviousIndexResult=on  ProcessOutOfRangeInput=Linear extrapolation  IndexDataType=sfix(16)  FractionDataType=sfix(16)  FractionScaling=2^0
  CX : Interpolation_n-D  NumberOfTableDimensions=3  Table=CX2  CheckIndexInCode=off  OutDataType=sfix(16)  OutScaling=2^0
  CY : Interpolation_n-D  NumberOfTableDimensions=3  Table=CY2  CheckIndexInCode=off  OutDataType=sfix(16)  OutScaling=2^0
  CZ : Interpolation_n-D  NumberOfTableDimensions=3  Table=CZ2  CheckIndexInCode=off  OutDataType=sfix(16)  OutScaling=2^0
  Cl : Interpolation_n-D  NumberOfTableDimensions=3  Table=Cl2  CheckIndexInCode=off  OutDataTypeMode=double  OutDataType=sfix(16)  OutScaling=2^0  OutDataTypeStr=double
  Cm : Interpolation_n-D  NumberOfTableDimensions=3  Table=Cm2  CheckIndexInCode=off  OutDataType=sfix(16)  OutScaling=2^0
  Cn : Interpolation_n-D  NumberOfTableDimensions=3  Table=Cn2  CheckIndexInCode=off  OutDataType=sfix(16)  OutScaling=2^0
  Demux : Demux  Outputs=2
  Mach Lookup : PreLookup  BreakpointsData=Machs  BeginIndexSearchUsingPreviousIndexResult=on  ProcessOutOfRangeInput=Linear extrapolation  IndexDataType=sfix(16)  FractionDataType=sfix(16)  FractionScaling=2^0
  Mux1 : Mux  Inputs=6
  Coeff : Outport  OutDataType=sfix(16)  OutScaling=2^0  InitialOutput=0
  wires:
  Demux/1 -> Alpha Lookup/1
  CX/1 -> Mux1/1, " CA"/1
  CY/1 -> Mux1/2, " Cy"/1
  CZ/1 -> Mux1/3, " CZ"/1
  Cl/1 -> Mux1/4, " Cl"/1
  Cm/1 -> Mux1/5, " Cm"/1
  Cn/1 -> Mux1/6, " Cn"/1
  Alpha Lookup/1 -> CX/1, CY/1, Cm/1, Cn/1, Cl/1, CZ/1
  Alpha Lookup/2 -> CX/2, CY/2, CZ/2, Cl/2, Cm/2, Cn/2
  Mach Lookup/1 -> CY/3, Cm/3, Cn/3, Cl/3, CZ/3, CX/3
  Mach Lookup/2 -> CY/4, Cm/4, Cn/4, Cl/4, CZ/4, CX/4
  Beta Lookup/1 -> CX/5, Cm/5, Cn/5, Cl/5, CZ/5, CY/5
  Beta Lookup/2 -> CX/6, CY/6, Cm/6, Cn/6, Cl/6, CZ/6
  Demux/2 -> Beta Lookup/1
  albet/1 -> Demux/1
  Mach/1 -> Mach Lookup/1
  Mux1/1 -> Coeff/1

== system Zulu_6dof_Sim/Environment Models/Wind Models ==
  note: Wind Disturbance Model (Shear, Gust, Turbulence)
  note: Air-Speed
  Ve : Inport  OutDataType=sfix(16)  OutScaling=2^0
  Altitude : Inport  Port=2  OutDataType=sfix(16)  OutScaling=2^0
  DCM : Inport  Port=3  OutDataType=sfix(16)  OutScaling=2^0
  Discrete Wind Gust Model - On : aerolibwind2/Discrete Wind Gust Model  SystemSampleTime=-1  units=English (Velocity in ft/s)  Gx=on  Gy=on  Gz=on  t_0=20  d_m=[120 120 80]  v_m=[3.5 3.0 3.0]*0
  Dot Product : DotProduct  OutDataType=sfix(16)  OutScaling=2^-10  SaturateOnIntegerOverflow=on
  Dryden Wind Turbulence Model  (Continuous (+q -r)) : aerolibwind2/Dryden Wind Turbulence Model  (Continuous (+q -r))  SystemSampleTime=-1  units=English (Velocity in ft/s)  spec=MIL-F-8785C  model=Continuous Dryden (+q -r)  W20=5  Wdeg=0  TurbProb=10^-2 - Light  L_high=533.4  Wingspan=4  ts=0.1  Seed=[23341 23342 23343 23344]  T_on=on
  Sum : Sum  Inputs=+++  OutDataType=sfix(16)  OutScaling=2^0
  V : Math  Operator=sqrt  OutDataType=sfix(16)  OutScaling=2^0
  V0 : ToWorkspace  VariableName=V0  SampleTime=-1  SaveFormat=Array
  Wind Shear Model : aerolibwind2/Wind Shear Model  SystemSampleTime=-1  units=English (Velocity in ft/s)  phase=Other  W_20=2  Wdeg=-50
  ug,vg,wg : Outport  OutDataType=sfix(16)  OutScaling=2^0
  pg,qg,rg : Outport  Port=2  OutDataType=sfix(16)  OutScaling=2^0
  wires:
  Dryden Wind Turbulence Model  (Continuous (+q -r))/1 -> Sum/2
  DCM/1 -> Wind Shear Model/2, Dryden Wind Turbulence Model  (Continuous (+q -r))/3
  Altitude/1 -> Dryden Wind Turbulence Model  (Continuous (+q -r))/1, Wind Shear Model/1
  Dot Product/1 -> V/1
  Ve/1 -> Dot Product/1, Dot Product/2
  V/1 -> Dryden Wind Turbulence Model  (Continuous (+q -r))/2, Discrete Wind Gust Model - On/1, [V0], V0/1
  Sum/1 -> ug,vg,wg/1
  Dryden Wind Turbulence Model  (Continuous (+q -r))/2 -> pg,qg,rg/1
  Discrete Wind Gust Model - On/1 -> Sum/3
  Wind Shear Model/1 -> Sum/1

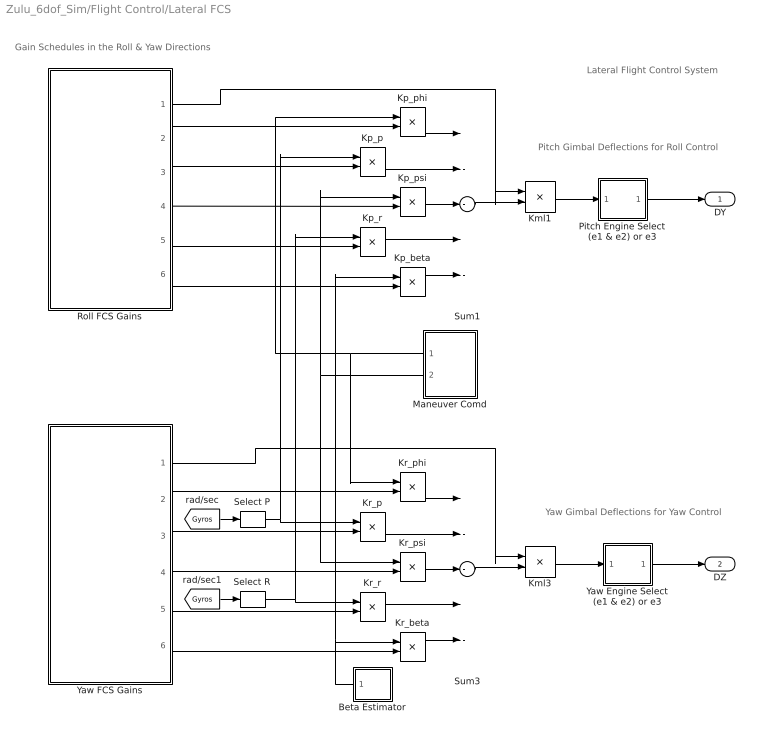
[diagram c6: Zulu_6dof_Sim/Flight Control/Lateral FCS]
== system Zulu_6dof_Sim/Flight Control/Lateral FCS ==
  note: Pitch Gimbal Deflections for Roll Control
  note: Lateral Flight Control System
  note: Yaw Gimbal Deflections for Yaw Control
  note: Gain Schedules in the Roll & Yaw Directions
  Beta Estimator : Subsystem
  Kml1 : Product  OutDataType=fixdt(1, 16)  OutScaling=2^0
  Kml3 : Product  OutDataType=fixdt(1, 16)  OutScaling=2^0
  Kp_beta : Product  OutDataType=fixdt(1, 16)  OutScaling=2^0
  Kp_p : Product  OutDataType=fixdt(1, 16)  OutScaling=2^0
  Kp_phi : Product  OutDataType=fixdt(1, 16)  OutScaling=2^0
  Kp_psi : Product  OutDataType=fixdt(1, 16)  OutScaling=2^0
  Kp_r : Product  OutDataType=fixdt(1, 16)  OutScaling=2^0
  Kr_beta : Product  OutDataType=fixdt(1, 16)  OutScaling=2^0
  Kr_p : Product  OutDataType=fixdt(1, 16)  OutScaling=2^0
  Kr_phi : Product  OutDataType=fixdt(1, 16)  OutScaling=2^0
  Kr_psi : Product  OutDataType=fixdt(1, 16)  OutScaling=2^0
  Kr_r : Product  OutDataType=fixdt(1, 16)  OutScaling=2^0
  Maneuver Comd : Subsystem
  Pitch Engine Select (e1 & e2) or e3 : Subsystem
  Roll FCS Gains : Subsystem  Tag=STV Subsys  LoadFcn=sigbuilder_block('load');  StartFcn=sigbuilder_block('start');  StopFcn=sigbuilder_block('stop');  ClipboardFcn=sigbuilder_block('clipboard');
  Select P : Selector  InputPortWidth=3  IndexOptions=Index vector (dialog)  Indices=[1]  OutputSizes=1
  Select R : Selector  InputPortWidth=3  IndexOptions=Index vector (dialog)  Indices=[3]  OutputSizes=1
  Sum1 : Sum  Inputs=-----  OutDataType=fixdt(1, 16)  OutScaling=2^0
  Sum3 : Sum  Inputs=-----  OutDataType=fixdt(1, 16)  OutScaling=2^0
  Yaw Engine Select (e1 & e2) or e3 : Subsystem
  Yaw FCS Gains : Subsystem  Tag=STV Subsys  LoadFcn=sigbuilder_block('load');  StartFcn=sigbuilder_block('start');  StopFcn=sigbuilder_block('stop');  ClipboardFcn=sigbuilder_block('clipboard');
  DY : Outport
  DZ : Outport  Port=2
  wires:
  Roll FCS Gains/2(Kp_phi) -> Kp_phi/2
  Roll FCS Gains/3(Kp_p) -> Kp_p/2
  Roll FCS Gains/4(Kp_psi) -> Kp_psi/2
  Roll FCS Gains/5(Kp_r) -> Kp_r/2
  Roll FCS Gains/6(Kp_beta) -> Kp_beta/2
  Sum1/1 -> Kml1/2
  Kr_phi/1 -> Sum3/1
  Kr_p/1 -> Sum3/2
  Kr_psi/1 -> Sum3/3
  Kr_beta/1 -> Sum3/5
  Kr_r/1 -> Sum3/4
  Yaw FCS Gains/2(Kr_phi) -> Kr_phi/2
  Yaw FCS Gains/3(Kr_p) -> Kr_p/2
  Yaw FCS Gains/4(Kr_psi) -> Kr_psi/2
  Yaw FCS Gains/5(Kr_r) -> Kr_r/2
  Yaw FCS Gains/6(Kr_beta) -> Kr_beta/2
  Sum3/1 -> Kml3/2
  Yaw FCS Gains/1(Kml3) -> Kml3/1
  Kp_p/1 -> Sum1/2
  Kp_psi/1 -> Sum1/3
  Kp_r/1 -> Sum1/4
  Kp_beta/1 -> Sum1/5
  Kp_phi/1 -> Sum1/1
  Kml3/1 -> Yaw Engine Select (e1 & e2) or e3/1("DZ ")
  Yaw Engine Select (e1 & e2) or e3/1(DZ) -> DZ/1
  Kml1/1 -> Pitch Engine Select (e1 & e2) or e3/1("DY ")
  Pitch Engine Select (e1 & e2) or e3/1(DY) -> DY/1
  Roll FCS Gains/1(Kml1) -> Kml1/1
  Select R/1 -> Kr_r/1, Kp_r/1
  Maneuver Comd/1(Phi-err) -> Kp_phi/1, Kr_phi/1
  Select P/1 -> Kr_p/1, Kp_p/1
  Maneuver Comd/2(Psi-err) -> Kr_psi/1, Kp_psi/1
  Beta Estimator/1(betest) -> Kr_beta/1, Kp_beta/1
  [Gyros] -> Select P/1
  [Gyros] -> Select R/1

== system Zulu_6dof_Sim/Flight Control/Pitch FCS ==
  note: Pitch Gimbal Deflections
  note: Pitch Flight Control System
  note: Vector
  note: Scalar
  note: Gain Schedules in the Longitudinal Directions
  Alpha Estimator : Subsystem
  Engine Select (e1 & e2) or e3 : Subsystem
  Guidance  Commands : Subsystem  Tag=STV Subsys  LoadFcn=sigbuilder_block('load');  StartFcn=sigbuilder_block('start');  StopFcn=sigbuilder_block('stop');  ClipboardFcn=sigbuilder_block('clipboard');
  Int : Integrator
  Kml2 : Product  OutDataType=fixdt(1, 16)  OutScaling=2^0
  Kq_alf : Product  OutDataType=fixdt(1, 16)  OutScaling=2^0
  Kq_gmi : Product  OutDataType=fixdt(1, 16)  OutScaling=2^0
  Kq_q : Product  OutDataType=fixdt(1, 16)  OutScaling=2^0
  Kq_the : Product  OutDataType=fixdt(1, 16)  OutScaling=2^0
  Pitch FCS Gains Desig Mod : Subsystem  Tag=STV Subsys  LoadFcn=sigbuilder_block('load');  StartFcn=sigbuilder_block('start');  StopFcn=sigbuilder_block('stop');  ClipboardFcn=sigbuilder_block('clipboard');
  Select Q : Selector  InputPortWidth=3  IndexOptions=Index vector (dialog)  Indices=[2]  OutputSizes=1
  Sum : Sum  Inputs=+-|  OutDataType=fixdt(1, 16)  OutScaling=2^0
  Sum1 : Sum  Inputs=|-+  OutDataType=fixdt(1, 16)  OutScaling=2^0
  Sum2 : Sum  Inputs=----  OutDataType=fixdt(1, 16)  OutScaling=2^0
  d2r : Gain  Gain=d2r  ParameterDataType=sfix(16)  ParameterScaling=2^0  OutDataType=sfix(16)  OutScaling=2^0
  "d2r " : Gain  Gain=d2r  ParameterDataType=sfix(16)  ParameterScaling=2^0  OutDataType=sfix(16)  OutScaling=2^0
  DY : Outport
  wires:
  Select Q/1 -> Kq_q/2
  [gamma] -> Sum1/2
  [theta] -> Sum/1
  Guidance  Commands/2(Gamma_cmd) -> "d2r "/1
  Sum/1 -> Kq_the/2
  Kq_the/1 -> Sum2/1
  Sum2/1 -> Kml2/2
  Pitch FCS Gains Desig Mod/1(Kml2) -> Kml2/1
  Kq_q/1 -> Sum2/3
  Pitch FCS Gains Desig Mod/3(Kq_gam_int) -> Kq_gmi/1
  d2r/1 -> Sum/2
  "d2r "/1 -> Sum1/1
  Sum1/1 -> Int/1
  Int/1 -> Kq_gmi/2
  Guidance  Commands/1(Theta_cmd) -> d2r/1
  Kq_gmi/1 -> Sum2/2
  Kq_alf/1 -> Sum2/4
  Pitch FCS Gains Desig Mod/2(Kq_theta) -> Kq_the/1
  Pitch FCS Gains Desig Mod/4(Kq_q) -> Kq_q/1
  Pitch FCS Gains Desig Mod/5(Kq_alpha) -> Kq_alf/1
  Kml2/1 -> Engine Select (e1 & e2) or e3/1("DY ")
  Engine Select (e1 & e2) or e3/1(DY) -> DY/1
  Alpha Estimator/1(alfest) -> Kq_alf/2
  [Gyros] -> Select Q/1

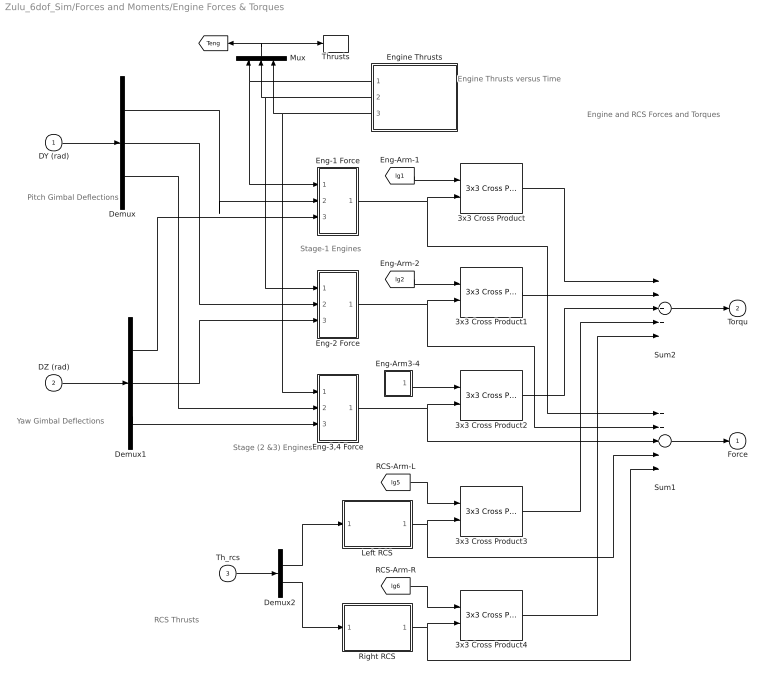
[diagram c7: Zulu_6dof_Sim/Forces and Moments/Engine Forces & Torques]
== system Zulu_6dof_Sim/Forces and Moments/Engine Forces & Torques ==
  note: Engine and RCS Forces and Torques
  note: RCS Thrusts
  note: Pitch Gimbal Deflections
  note: Yaw Gimbal Deflections
  note: Engine Thrusts versus Time
  note: Stage-1 Engines
  note: Stage (2 &3) Engines
  DY (rad) : Inport  OutDataType=sfix(16)  OutScaling=2^0
  DZ (rad) : Inport  Port=2  OutDataType=sfix(16)  OutScaling=2^0
  Th_rcs : Inport  Port=3  OutDataType=sfix(16)  OutScaling=2^0
  3x3 Cross Product{,1..4} (5 alike) : aerolibutil/3x3 Cross Product  SystemSampleTime=-1
  Demux : Demux  Outputs=3
  Demux1 : Demux  Outputs=3
  Demux2 : Demux  Outputs=2
  Eng-1 Force : Subsystem
  Eng-2 Force : Subsystem
  Eng-3,4 Force : Subsystem
  Eng-Arm3-4 : Subsystem
  Engine Thrusts : Subsystem  Tag=STV Subsys  LoadFcn=sigbuilder_block('load');  StartFcn=sigbuilder_block('start');  StopFcn=sigbuilder_block('stop');  ClipboardFcn=sigbuilder_block('clipboard');
  Left RCS : Subsystem
  Mux : Mux  Inputs=3
  Right RCS : Subsystem
  Sum1 : Sum  Inputs=+++++  OutDataType=fixdt(1, 16)  OutScaling=2^0
  Sum2 : Sum  Inputs=+++++  OutDataType=fixdt(1, 16)  OutScaling=2^0
  Thrusts : ToWorkspace  VariableName=Teng  SampleTime=-1  SaveFormat=Array
  Force : Outport  OutDataType=sfix(16)  OutScaling=2^0  InitialOutput=0
  Torqu : Outport  Port=2  OutDataType=sfix(16)  OutScaling=2^0  InitialOutput=0
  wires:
  Sum1/1 -> Force/1
  3x3 Cross Product2/1 -> Sum2/3
  3x3 Cross Product/1 -> Sum2/1
  3x3 Cross Product1/1 -> Sum2/2
  Eng-Arm3-4/1(lg3) -> 3x3 Cross Product2/1
  Eng-3,4 Force/1(F1) -> 3x3 Cross Product2/2, Sum1/3
  [lg2] -> 3x3 Cross Product1/1
  Eng-2 Force/1(F1) -> Sum1/2, 3x3 Cross Product1/2
  [lg1] -> 3x3 Cross Product/1
  Demux1/3 -> Eng-3,4 Force/3(dz)
  Demux/3 -> Eng-3,4 Force/2(dy)
  Demux1/2 -> Eng-2 Force/3(dz)
  Demux1/1 -> Eng-1 Force/3(dz)
  Eng-1 Force/1(F1) -> Sum1/1, 3x3 Cross Product/2
  DZ (rad)/1 -> Demux1/1
  DY (rad)/1 -> Demux/1
  Engine Thrusts/1(Thrust-1) -> Eng-1 Force/1(Thrust), Mux/1
  Engine Thrusts/2(Thrust-2) -> Eng-2 Force/1(Thrust), Mux/2
  Left RCS/1(FL) -> 3x3 Cross Product3/2, Sum1/4
  [lg5] -> 3x3 Cross Product3/1
  Demux2/2 -> Right RCS/1(Thrust)
  Right RCS/1(FL) -> 3x3 Cross Product4/2, Sum1/5
  [lg6] -> 3x3 Cross Product4/1
  3x3 Cross Product3/1 -> Sum2/4
  3x3 Cross Product4/1 -> Sum2/5
  Sum2/1 -> Torqu/1
  Th_rcs/1 -> Demux2/1
  Demux2/1 -> Left RCS/1(Thrust)
  Demux/2 -> Eng-2 Force/2(dy)
  Demux/1 -> Eng-1 Force/2(dy)
  Engine Thrusts/3(Thrust-3) -> Eng-3,4 Force/1(Thrust), Mux/3
  Mux/1 -> Thrusts/1, [Teng]

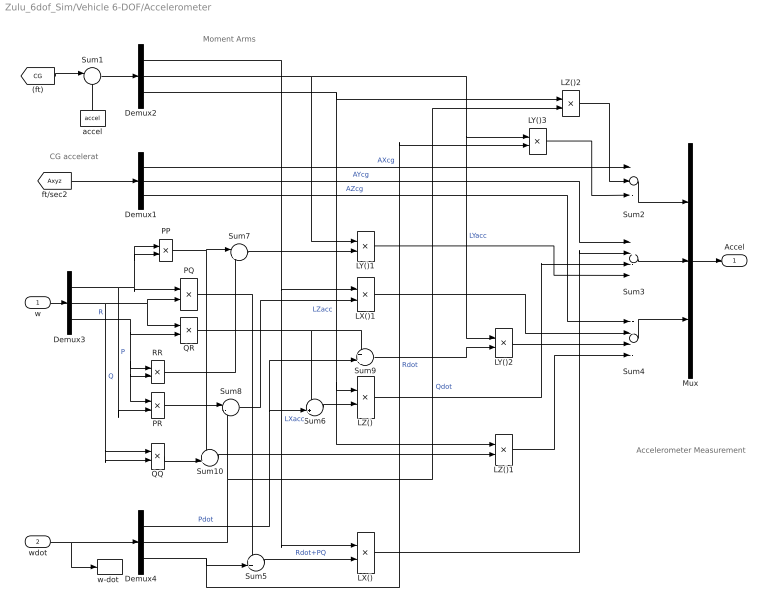
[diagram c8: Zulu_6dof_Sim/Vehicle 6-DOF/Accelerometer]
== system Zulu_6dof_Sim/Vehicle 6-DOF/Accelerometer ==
  note: CG accelerat
  note: Moment Arms
  note: Accelerometer Measurement
  w : Inport
  wdot : Inport  Port=2
  Demux{1..4} (4 alike) : Demux  Outputs=3
  LX() : Product  OutDataType=fixdt(1, 16)  OutScaling=2^0
  LX()1 : Product  OutDataType=fixdt(1, 16)  OutScaling=2^0
  LY()1 : Product  OutDataType=fixdt(1, 16)  OutScaling=2^0
  LY()2 : Product  OutDataType=fixdt(1, 16)  OutScaling=2^0
  LY()3 : Product  OutDataType=fixdt(1, 16)  OutScaling=2^0
  LZ() : Product  OutDataType=fixdt(1, 16)  OutScaling=2^0
  LZ()1 : Product  OutDataType=fixdt(1, 16)  OutScaling=2^0
  LZ()2 : Product  OutDataType=fixdt(1, 16)  OutScaling=2^0
  Mux : Mux  Inputs=3
  PP : Product  OutDataType=fixdt(1, 16)  OutScaling=2^0
  PQ : Product  OutDataType=fixdt(1, 16)  OutScaling=2^0
  PR : Product  OutDataType=fixdt(1, 16)  OutScaling=2^0
  QQ : Product  OutDataType=fixdt(1, 16)  OutScaling=2^0
  QR : Product  OutDataType=fixdt(1, 16)  OutScaling=2^0
  RR : Product  OutDataType=fixdt(1, 16)  OutScaling=2^0
  Sum1 : Sum  Inputs=|-+  OutDataType=fixdt(1, 16)  OutScaling=2^0
  Sum10 : Sum  Inputs=++|  OutDataType=fixdt(1, 16)  OutScaling=2^0
  Sum2 : Sum  Inputs=++-  OutDataType=fixdt(1, 16)  OutScaling=2^0
  Sum3 : Sum  Inputs=++--  OutDataType=fixdt(1, 16)  OutScaling=2^0
  Sum4 : Sum  Inputs=+---  OutDataType=fixdt(1, 16)  OutScaling=2^0
  Sum5 : Sum  Inputs=++|  OutDataType=fixdt(1, 16)  OutScaling=2^0
  Sum6 : Sum  Inputs=-+|  OutDataType=fixdt(1, 16)  OutScaling=2^0
  Sum7 : Sum  Inputs=|++  OutDataType=fixdt(1, 16)  OutScaling=2^0
  Sum8 : Sum  Inputs=|-+  OutDataType=fixdt(1, 16)  OutScaling=2^0
  Sum9 : Sum  Inputs=++|  OutDataType=fixdt(1, 16)  OutScaling=2^0
  accel : Constant  Value=accel  OutDataType=fixdt(1, 16)  OutScaling=2^0
  "w-dot " : ToWorkspace  VariableName=Wdot  SampleTime=-1  SaveFormat=Array
  Accel : Outport
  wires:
  accel/1 -> Sum1/2
  [CG] -> Sum1/1
  Sum1/1 -> Demux2/1
  w/1 -> Demux3/1
  wdot/1 -> Demux4/1, "w-dot "/1
  Demux2/1 -> LX()/1, LX()1/1  "LXacc"
  Demux2/2 -> LY()1/1, LY()2/1, LY()3/1  "LYacc"
  Demux2/3 -> LZ()/1, LZ()1/1, LZ()2/1  "LZacc"
  Demux3/1 -> PQ/1, PP/2, PP/1, PR/2  "P"
  Demux3/2 -> PQ/2, QR/1, QQ/1, QQ/2  "Q"
  Demux3/3 -> QR/2, RR/1, RR/2, PR/1  "R"
  Demux4/1 -> Sum6/2, Sum9/2  "Pdot"
  Demux4/2 -> Sum8/2, LZ()2/2  "Qdot"
  Demux4/3 -> Sum5/2, LY()3/2  "Rdot"
  [Axyz] -> Demux1/1
  Demux1/1 -> Sum2/1  "AXcg"
  Sum2/1 -> Mux/1
  Sum3/1 -> Mux/2
  Demux1/2 -> Sum3/1  "AYcg"
  Sum4/1 -> Mux/3
  Demux1/3 -> Sum4/1  "AZcg"
  PQ/1 -> Sum5/1
  Sum5/1 -> LX()/2  "Rdot+PQ"
  LX()/1 -> Sum3/2
  QR/1 -> Sum6/1, Sum9/1
  Sum6/1 -> LZ()/2
  LZ()/1 -> Sum3/3
  PP/1 -> Sum7/1, Sum10/1
  RR/1 -> Sum7/2
  Sum7/1 -> LY()1/2
  LY()1/1 -> Sum3/4
  PR/1 -> Sum8/1
  Sum8/1 -> LX()1/2
  LX()1/1 -> Sum4/2
  Sum9/1 -> LY()2/2
  LY()2/1 -> Sum4/3
  QQ/1 -> Sum10/2
  Sum10/1 -> LZ()1/2
  LZ()1/1 -> Sum4/4
  LZ()2/1 -> Sum2/2
  LY()3/1 -> Sum2/3
  Mux/1 -> Accel/1

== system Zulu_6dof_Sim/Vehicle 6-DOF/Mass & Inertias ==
  note: Mass Properties versus Time
  note: CG and Moment Arm Calculations
  note: Moments of Inertia Matrix
  CG Variat : Subsystem
  Create Moments  of Inertia Matrix : aerolibutil/Create 3x3 Matrix  SystemSampleTime=-1
  Mass : ToWorkspace  VariableName=mass  SampleTime=-1  SaveFormat=Array
  Mass vs Time : Subsystem  Tag=STV Subsys  LoadFcn=sigbuilder_block('load');  StartFcn=sigbuilder_block('start');  StopFcn=sigbuilder_block('stop');  ClipboardFcn=sigbuilder_block('clipboard');
  Moments of Inertia : Subsystem
  mass : Outport
  Inert : Outport  Port=2
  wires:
  Mass vs Time/1(Mass (slg)) -> Moments of Inertia/1(mass), CG Variat/1(m), [mass], mass/1, Mass/1
  Create Moments  of Inertia Matrix/1 -> Inert/1
  Moments of Inertia/6(Iyz) -> Create Moments  of Inertia Matrix/6, Create Moments  of Inertia Matrix/8
  Moments of Inertia/5(Ixz) -> Create Moments  of Inertia Matrix/7, Create Moments  of Inertia Matrix/3
  Moments of Inertia/2(Iyy) -> Create Moments  of Inertia Matrix/5
  Moments of Inertia/3(Izz) -> Create Moments  of Inertia Matrix/9
  Moments of Inertia/1(Ixx) -> Create Moments  of Inertia Matrix/1
  Moments of Inertia/4(Ixy) -> Create Moments  of Inertia Matrix/4, Create Moments  of Inertia Matrix/2

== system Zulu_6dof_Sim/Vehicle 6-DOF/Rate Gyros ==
  note: Rate Gyro Measurement
  w : Inport
  Demux3 : Demux  Outputs=3
  Gyro1 : TransferFcn  Numerator=[100]  Denominator=[1 100]
  Gyro2 : TransferFcn  Numerator=[100]  Denominator=[1 100]
  Gyro3 : TransferFcn  Numerator=[100]  Denominator=[1 100]
  Mux : Mux  Inputs=3
  w-body : ToWorkspace  VariableName=Wb  SampleTime=-1  SaveFormat=Array
  Gyro : Outport
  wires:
  w/1 -> Demux3/1, w-body/1
  Mux/1 -> Gyro/1
  Gyro2/1 -> Mux/1
  Gyro1/1 -> Mux/2
  Gyro3/1 -> Mux/3
  Demux3/2 -> Gyro1/1  "Q"
  Demux3/1 -> Gyro2/1  "P"
  Demux3/3 -> Gyro3/1  "R"

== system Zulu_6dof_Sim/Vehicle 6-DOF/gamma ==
  note: Flight Path Angle, Direction, CrossRange, DownRange
  Ve : Inport
  -1 : Gain  Gain=-1  ParameterDataType=sfix(16)  ParameterScaling=2^0  OutDataType=sfix(16)  OutScaling=2^0
  57.2 : Gain  Gain=180/pi  ParameterDataType=sfix(16)  ParameterScaling=2^0  OutDataType=sfix(16)  OutScaling=2^0
  Int1 : Integrator
  Int2 : Integrator
  "Ve " : Scope
  Vearth : ToWorkspace  VariableName=Ve  SampleTime=-1  SaveFormat=Array
  Vx : Selector  InputPortWidth=3  IndexOptions=Index vector (dialog)  Indices=[1]  OutputSizes=1
  Vy : Selector  InputPortWidth=3  IndexOptions=Index vector (dialog)  Indices=[2]  OutputSizes=1
  Vz : Selector  InputPortWidth=3  IndexOptions=Index vector (dialog)  Indices=[3]  OutputSizes=1
  atan : Trigonometry  Operator=atan2
  atan1 : Trigonometry  Operator=atan2
  cross range : ToWorkspace  VariableName=xrng  SampleTime=-1  SaveFormat=Array
  direction : ToWorkspace  VariableName=direct  SampleTime=-1  SaveFormat=Array
  down-range : ToWorkspace  VariableName=dnr  SampleTime=-1  SaveFormat=Array
  "gam " : Scope
  gama : ToWorkspace  VariableName=gama  SampleTime=-1  SaveFormat=Array
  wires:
  Vz/1 -> -1/1
  Vx/1 -> atan/2, atan1/2, Int2/1
  atan/1 -> 57.2/1, [gamma]
  57.2/1 -> "gam "/1, gama/1
  Ve/1 -> Vx/1, Vy/1, "Ve "/1, Vz/1, Vearth/1
  Vy/1 -> atan1/1, Int1/1
  atan1/1 -> [direct], direction/1
  -1/1 -> atan/1
  Int1/1 -> cross range/1
  Int2/1 -> [dnr], down-range/1

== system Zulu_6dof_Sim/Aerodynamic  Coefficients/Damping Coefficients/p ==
  Alpha : Inport  OutDataType=sfix(16)  OutScaling=2^0
  Constant1 : Constant  Value=0  OutDataType=sfix(16)  OutScaling=2^0
  Mux1 : Mux  Inputs=6
  grd : Terminator
  C : Outport
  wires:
  Mux1/1 -> C/1
  Constant1/1 -> Mux1/6, Mux1/5, Mux1/4, Mux1/3, Mux1/2, Mux1/1
  Alpha/1 -> grd/1

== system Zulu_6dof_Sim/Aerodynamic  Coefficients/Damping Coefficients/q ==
  Alpha : Inport  OutDataType=sfix(16)  OutScaling=2^0
  Constant1 : Constant  Value=0  OutDataType=sfix(16)  OutScaling=2^0
  Mux1 : Mux  Inputs=6
  grd : Terminator
  C : Outport
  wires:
  Mux1/1 -> C/1
  Constant1/1 -> Mux1/6, Mux1/5, Mux1/4, Mux1/3, Mux1/2, Mux1/1
  Alpha/1 -> grd/1

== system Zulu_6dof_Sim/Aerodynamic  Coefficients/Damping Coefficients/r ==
  Alpha : Inport  OutDataType=sfix(16)  OutScaling=2^0
  Constant1 : Constant  Value=0  OutDataType=sfix(16)  OutScaling=2^0
  Mux1 : Mux  Inputs=6
  grd : Terminator
  C : Outport
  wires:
  Mux1/1 -> C/1
  Constant1/1 -> Mux1/6, Mux1/5, Mux1/4, Mux1/3, Mux1/2, Mux1/1
  Alpha/1 -> grd/1

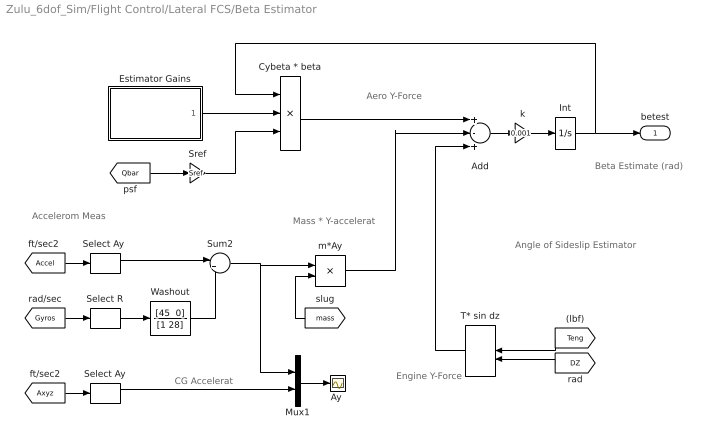
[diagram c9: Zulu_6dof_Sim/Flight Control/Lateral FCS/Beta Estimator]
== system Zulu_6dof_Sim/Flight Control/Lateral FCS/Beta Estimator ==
  note: Angle of Sideslip Estimator
  note: Engine Y-Force
  note: Aero Y-Force
  note: Mass * Y-accelerat
  note: Beta Estimate (rad)
  note: Accelerom Meas
  note: CG Accelerat
  Add : Sum  Inputs=+-+  OutDataType=fixdt(1, 16)  OutScaling=2^-10
  "Ay " : Scope
  Cybeta * beta : Product  Inputs=3  OutDataType=fixdt(1, 16)  OutScaling=2^0
  Estimator Gains : Subsystem  Tag=STV Subsys  LoadFcn=sigbuilder_block('load');  StartFcn=sigbuilder_block('start');  StopFcn=sigbuilder_block('stop');  ClipboardFcn=sigbuilder_block('clipboard');
  Int : Integrator
  Mux1 : Mux  Inputs=2
  Select Ay : Selector  InputPortWidth=3  IndexOptions=Index vector (dialog)  Indices=[2]  OutputSizes=1
  "Select Ay " : Selector  InputPortWidth=3  IndexOptions=Index vector (dialog)  Indices=[2]  OutputSizes=1
  Select R : Selector  InputPortWidth=3  IndexOptions=Index vector (dialog)  Indices=[3]  OutputSizes=1
  Sref : Gain  Gain=Sref  ParameterDataType=sfix(16)  ParameterScaling=2^0  OutDataType=sfix(16)  OutScaling=2^0
  Sum2 : Sum  Inputs=|+-  OutDataType=fixdt(1, 16)  OutScaling=2^0
  T* sin dz : DotProduct  OutDataType=fixdt(1, 16)  OutScaling=2^-10
  Washout : TransferFcn  Numerator="[45  0]"  Denominator=[1 28]
  k : Gain  Gain=0.001  ParameterDataType=sfix(16)  ParameterScaling=2^0  OutDataType=sfix(16)  OutScaling=2^0
  m*Ay : Product  OutDataType=fixdt(1, 16)  OutScaling=2^0
  betest : Outport
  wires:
  [DZ] -> T* sin dz/2
  [Teng] -> T* sin dz/1
  [mass] -> m*Ay/2
  [Qbar] -> Sref/1
  Int/1 -> Cybeta * beta/1, betest/1
  Estimator Gains/1(Cy_beta) -> Cybeta * beta/2
  Cybeta * beta/1 -> Add/1
  Add/1 -> k/1
  m*Ay/1 -> Add/2
  T* sin dz/1 -> Add/3
  k/1 -> Int/1
  Sref/1 -> Cybeta * beta/3
  [Axyz] -> Select Ay/1
  [Gyros] -> Select R/1
  Select R/1 -> Washout/1
  [Accel] -> "Select Ay "/1
  "Select Ay "/1 -> Sum2/1
  Washout/1 -> Sum2/2
  Mux1/1 -> "Ay "/1
  Sum2/1 -> m*Ay/1, Mux1/1
  Select Ay/1 -> Mux1/2

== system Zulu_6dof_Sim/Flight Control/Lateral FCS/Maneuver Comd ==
  note: Direction Error
  note: Becomes Roll & Yaw Commands
  note: Flight Direction Feedback
  note: Lateral Guidance
  Direction Command : Subsystem  Tag=STV Subsys  LoadFcn=sigbuilder_block('load');  StartFcn=sigbuilder_block('start');  StopFcn=sigbuilder_block('stop');  ClipboardFcn=sigbuilder_block('clipboard');
  Int : Integrator
  Kphi : Gain  Gain=5  ParameterDataType=sfix(16)  ParameterScaling=2^0  OutDataType=sfix(16)  OutScaling=2^0
  Kpsi : Gain  Gain=10  ParameterDataType=sfix(16)  ParameterScaling=2^0  OutDataType=sfix(16)  OutScaling=2^0
  Sum : Sum  Inputs=-+|  OutDataType=fixdt(1, 16)  OutScaling=2^0
  Sum1 : Sum  Inputs=+-|  OutDataType=fixdt(1, 16)  OutScaling=2^0
  Sum2 : Sum  Inputs=|-+  OutDataType=fixdt(1, 16)  OutScaling=2^0
  Sum3 : Sum  Inputs=|++  OutDataType=fixdt(1, 16)  OutScaling=2^0
  d2r : Gain  Gain=d2r  ParameterDataType=sfix(16)  ParameterScaling=2^0  OutDataType=sfix(16)  OutScaling=2^0
  ki : Gain  Gain=0.1  ParameterDataType=sfix(16)  ParameterScaling=2^0  OutDataType=sfix(16)  OutScaling=2^0
  Phi-err : Outport
  Psi-err : Outport  Port=2
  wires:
  Direction Command/1(Direct Cmd) -> d2r/1
  [phi] -> Sum1/1
  [psi] -> Sum2/2
  Sum1/1 -> Phi-err/1
  Sum2/1 -> Psi-err/1
  Kpsi/1 -> Sum2/1
  d2r/1 -> Sum/2
  Kphi/1 -> Sum1/2
  Sum/1 -> Sum3/1, Int/1
  Sum3/1 -> Kphi/1, Kpsi/1
  Int/1 -> ki/1
  ki/1 -> Sum3/2
  [direct] -> Sum/1

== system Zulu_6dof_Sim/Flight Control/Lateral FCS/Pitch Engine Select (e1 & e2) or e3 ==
  note: Stage-1
  note: Stage-2
  note: Command Left & Right Engines Differentially in Pitch for Roll Control Only During Stage-1
  "DY " : Inport
  -1 : Gain  Gain=-1  ParameterDataType=sfix(16)  ParameterScaling=2^0  OutDataType=sfix(16)  OutScaling=2^0
  Clock : Clock
  Mux : Mux  Inputs=3
  Switch : Switch  Threshold=Tstg  OutDataType=fixdt(1, 16)  OutScaling=2^0
  grd : Ground
  DY : Outport
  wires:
  Clock/1 -> Switch/2
  "DY "/1 -> Switch/3
  Switch/1 -> Mux/1, -1/1
  grd/1 -> Switch/1, Mux/3
  Mux/1 -> DY/1
  -1/1 -> Mux/2

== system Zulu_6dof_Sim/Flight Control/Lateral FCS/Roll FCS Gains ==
  Demux : Demux  Tag=STV Demux  Outputs=6
  FromWs : FromWorkspace  Tag=STV FromWs  VariableName=tuvar  SampleTime=0  SigBuilderData=DataTag4  VnvData=DataTag5
  Kml1 : Outport  Tag=STV Outport
  Kp_phi : Outport  Tag=STV Outport  Port=2
  Kp_p : Outport  Tag=STV Outport  Port=3
  Kp_psi : Outport  Tag=STV Outport  Port=4
  Kp_r : Outport  Tag=STV Outport  Port=5
  Kp_beta : Outport  Tag=STV Outport  Port=6
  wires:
  FromWs/1 -> Demux/1
  Demux/1 -> Kml1/1
  Demux/2 -> Kp_phi/1
  Demux/3 -> Kp_p/1
  Demux/4 -> Kp_psi/1
  Demux/5 -> Kp_r/1
  Demux/6 -> Kp_beta/1

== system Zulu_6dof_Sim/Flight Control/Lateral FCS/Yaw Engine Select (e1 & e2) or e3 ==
  note: Stage-1
  note: Stage-2
  note: Deflect Left & Right Engines in Yaw for Yaw Control During Stage-1
  note: Otherwise, During Stage-2 and 3, Deflect the Middle Engine in Yaw for Yaw Control
  "DZ " : Inport
  Clock : Clock
  Mux : Mux  Inputs=3
  Switch : Switch  Threshold=Tstg  OutDataType=fixdt(1, 16)  OutScaling=2^0
  Switch1 : Switch  Threshold=Tstg  OutDataType=fixdt(1, 16)  OutScaling=2^0
  grd : Ground
  DZ : Outport
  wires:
  Clock/1 -> Switch/2, Switch1/2
  "DZ "/1 -> Switch/3, Switch1/1
  Switch/1 -> Mux/1, Mux/2
  Switch1/1 -> Mux/3
  grd/1 -> Switch1/3, Switch/1
  Mux/1 -> DZ/1
